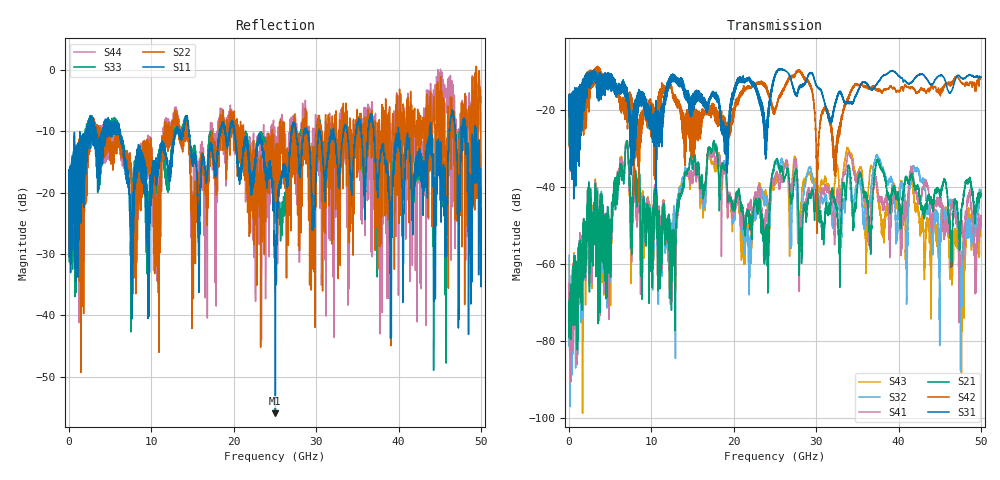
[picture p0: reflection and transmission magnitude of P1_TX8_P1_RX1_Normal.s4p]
!Keysight Technologies,N5225B,MY57041031,A.13.20.10
!Date: Friday, May 31, 2019 11:14:28
!Correction: S11(Full 4 Port(1,2,3,4))
!S12(Full 4 Port(1,2,3,4))
!S13(Full 4 Port(1,2,3,4))
!S14(Full 4 Port(1,2,3,4))
!S21(Full 4 Port(1,2,3,4))
!S22(Full 4 Port(1,2,3,4))
!S23(Full 4 Port(1,2,3,4))
!S24(Full 4 Port(1,2,3,4))
!S31(Full 4 Port(1,2,3,4))
!S32(Full 4 Port(1,2,3,4))
!S33(Full 4 Port(1,2,3,4))
!S34(Full 4 Port(1,2,3,4))
!S41(Full 4 Port(1,2,3,4))
!S42(Full 4 Port(1,2,3,4))
!S43(Full 4 Port(1,2,3,4))
!S44(Full 4 Port(1,2,3,4))
!S4P File: Measurements: <S11,S12,S13,S14>,
!<S21,S22,S23,S24>,
!<S31,S32,S33,S34>,
!<S41,S42,S43,S44>:
# Hz S  dB  R 50.0
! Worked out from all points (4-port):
!   5000 points, 10 MHz to 50 GHz, reference 50 ohm
!   strongest paths, dB at 10 MHz, 12.51 GHz, 25.01 GHz, 37.51 GHz, 50 GHz:
!     S31: -19.7, -10.8, -11.0, -12.6, -11.3
!     S42: -19.3, -14.7, -19.8, -15.0, -11.3
!     S21: -78.9, -51.2, -33.6, -33.0, -42.2
!     S41: -65.0, -55.6, -37.3, -41.4, -47.3
!     S32: -57.6, -50.4, -33.5, -32.2, -41.0
!     S43: -59.7, -52.8, -39.4, -43.6, -48.0
!   lowest |S11| = -55.9 dB at 25.05 GHz (marker M1), VSWR 1.00, Z = 49.9 + j0.0572 ohm
!   |S11| at or under -10 dB: 6.192 GHz to 12.89 GHz (6.696 GHz wide, 70.2 % of centre); 20.1 GHz to 26.99 GHz (6.893 GHz wide, 29.3 % of centre); 40 GHz to 43.77 GHz (3.764 GHz wide, 8.99 % of centre)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
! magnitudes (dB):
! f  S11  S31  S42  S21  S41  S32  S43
! 10 MHz  -19.5  -19.7  -19.3  -78.9  -65.0  -57.6  -59.7
! 7.01 GHz  -16.0  -16.1  -20.8  -28.8  -28.9  -28.3  -28.6
! 12.67 GHz  -12.6  -10.8  -16.4  -54.2  -54.2  -47.2  -47.8
! 25.05 GHz  -55.9  -10.5  -19.8  -33.4  -37.1  -33.4  -39.1
! 41.88 GHz  -20.3  -11.8  -14.4  -39.6  -38.9  -34.8  -43.4
! 47.6 GHz  -12.1  -11.6  -12.8  -48.2  -47.9  -65.8  -64.0
! 50 GHz  -22.5  -11.3  -11.3  -42.2  -47.3  -41.0  -48.0
